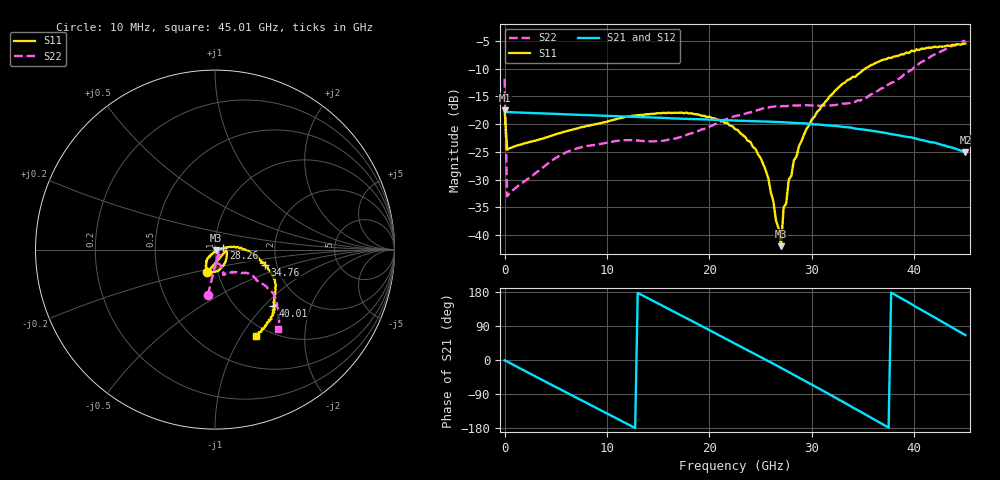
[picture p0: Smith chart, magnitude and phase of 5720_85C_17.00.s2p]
! Device:  ADRF5720
! Description: 0.5dB LSB GaAs MMIC 6-bit Digital Attenuator
! Frequency:  0.000009 -  40 GHz
! Ports:
!	RF1	= Port 1
!	RF2	= Port 2
! Vdd:  3.3 Volt
! Vss:  -3.3 Volt
! Control:  0/3.3 Volt
! State:  17.00 dB attenuation
! Data:  The device was measured using G-S-G Probes on a matrix board.
!  Data was collected using an calibrated 4 port network analyzer.
!  The reference plane for this measurement is at the launchers.
! Note:  Analog Devices supplies this data as a sample of measured data
!  for this product.  Your particular data for this product may vary.
!  Data was taken at 85 degrees C.
!  Analog Devices reserves the right to change this data at anytime.
# GHZ S DB R 45.0
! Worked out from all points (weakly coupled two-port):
!   181 points, 10 MHz to 45.01 GHz, reference 45 ohm
!   highest |S21| = -17.52 dB at 10 MHz (marker M1); lowest = -25.0 dB at 45.01 GHz (marker M2)
!   lowest |S11| = -42.0 dB at 27.01 GHz (marker M3), VSWR 1.02, Z = 45.6 - j0.431 ohm
!   |S11| at or under -10 dB: start of sweep to 35.24 GHz
!   |S22| runs from -33.0 to -4.9 dB; largest |S21 - S12| = 0.00065
!   S11 on the Smith chart (normalised r, x): 10 MHz: 0.89, -0.23; 28.26 GHz: 1.10, +0.02; 34.76 GHz: 1.73, -0.33; 40.01 GHz: 1.43, -1.13; 45.01 GHz: 0.86, -1.16
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0.01  -17.49 -108.6  -17.52 -1.2  -17.51 -1.2  -11.84 -98.9
0.26  -24.60 -9.0  -17.82 -3.9  -17.81 -3.9  -33.01 -21.9
5.01  -21.84 -38.7  -18.16 -71.3  -18.14 -71.3  -26.09 -67.8
7.76  -20.48 -56.6  -18.35 -109.8  -18.34 -109.7  -24.03 -82.9
15.26  -18.04 -94.8  -18.85 145.4  -18.84 145.6  -23.01 -87.0
20.01  -18.64 -113.3  -19.18 78.8  -19.17 79.0  -20.45 -70.2
22.76  -21.04 -122.7  -19.37 40.1  -19.35 40.2  -18.46 -68.8
24.51  -24.44 -128.1  -19.48 15.3  -19.47 15.5  -17.58 -70.5
25.51  -28.33 -123.7  -19.53 0.9  -19.51 1.2  -17.03 -71.4
26.26  -33.94 -115.9  -19.59 -9.9  -19.57 -9.7  -16.86 -70.9
27.01  -41.99 -36.4  -19.64 -20.9  -19.62 -20.6  -16.79 -70.6
27.26  -35.01 -11.8  -19.67 -24.6  -19.66 -24.3  -16.74 -71.3
27.51  -34.30 5.1  -19.70 -28.2  -19.69 -27.9  -16.78 -70.7
27.76  -30.01 5.1  -19.73 -31.8  -19.71 -31.5  -16.66 -71.5
28.01  -29.33 9.7  -19.76 -35.5  -19.75 -35.2  -16.71 -71.1
28.26  -26.49 9.8  -19.78 -39.0  -19.77 -38.8  -16.62 -71.6
30.26  -18.69 5.7  -20.02 -68.5  -20.00 -68.3  -16.74 -69.4
32.26  -14.02 -4.5  -20.30 -98.5  -20.28 -98.2  -16.57 -62.4
34.76  -10.69 -17.4  -20.90 -136.4  -20.88 -136.1  -15.74 -49.7
37.76  -8.05 -32.0  -21.80 177.8  -21.78 178.1  -12.55 -35.7
40.01  -6.89 -44.1  -22.53 143.0  -22.51 143.4  -9.79 -35.9
45.01  -5.47 -64.8  -25.05 65.8  -25.01 66.2  -4.92 -51.6
